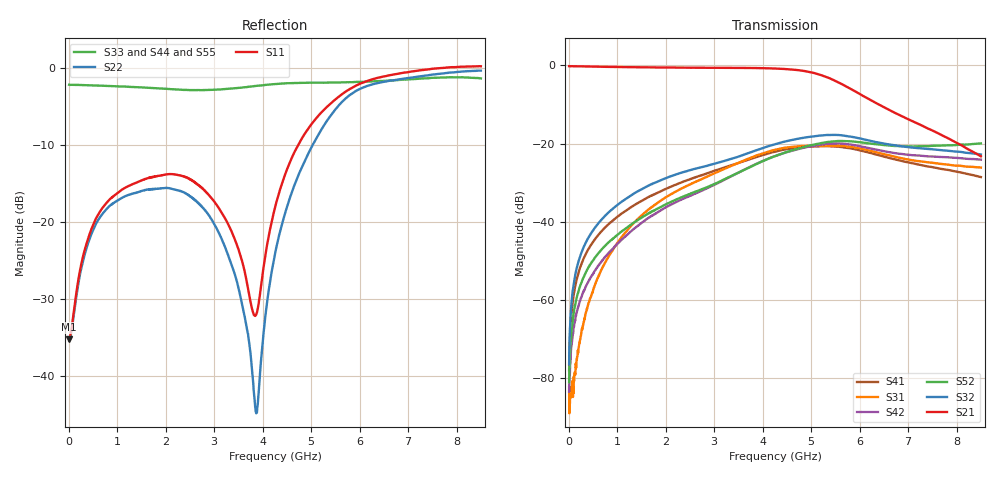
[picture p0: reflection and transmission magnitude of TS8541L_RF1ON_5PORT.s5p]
! Created with skrf (http://scikit-rf.org).
# Hz S RI R 50.0
!freq ReS11 ImS11 ReS12 ImS12 ReS13 ImS13
! ReS14 ImS14 ReS15 ImS15
! ReS21 ImS21 ReS22 ImS22 ReS23 ImS23
! ReS24 ImS24 ReS25 ImS25
! ReS31 ImS31 ReS32 ImS32 ReS33 ImS33
! ReS34 ImS34 ReS35 ImS35
! ReS41 ImS41 ReS42 ImS42 ReS43 ImS43
! ReS44 ImS44 ReS45 ImS45
! ReS51 ImS51 ReS52 ImS52 ReS53 ImS53
! ReS54 ImS54 ReS55 ImS55
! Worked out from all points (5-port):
!   1601 points, 10 MHz to 8.5 GHz, reference 50 ohm
!   strongest paths, dB at 10 MHz, 2.132 GHz, 4.255 GHz, 6.378 GHz, 8.5 GHz:
!     S21: -0.2, -0.5, -0.8, -9.9, -23.2
!     S32: -76.5, -28.2, -20.2, -19.7, -22.8
!     S52: -81.1, -34.8, -23.2, -20.2, -19.9
!     S42: -83.5, -35.5, -23.2, -21.6, -24.1
!     S31: -82.3, -32.8, -21.6, -22.3, -26.1
!     S41: -78.1, -30.9, -22.1, -22.9, -28.6
!   lowest |S11| = -35.2 dB at 10 MHz (marker M1), VSWR 1.04, Z = 51.8 - j0.199 ohm
!   |S11| at or under -10 dB: start of sweep to 4.732 GHz
